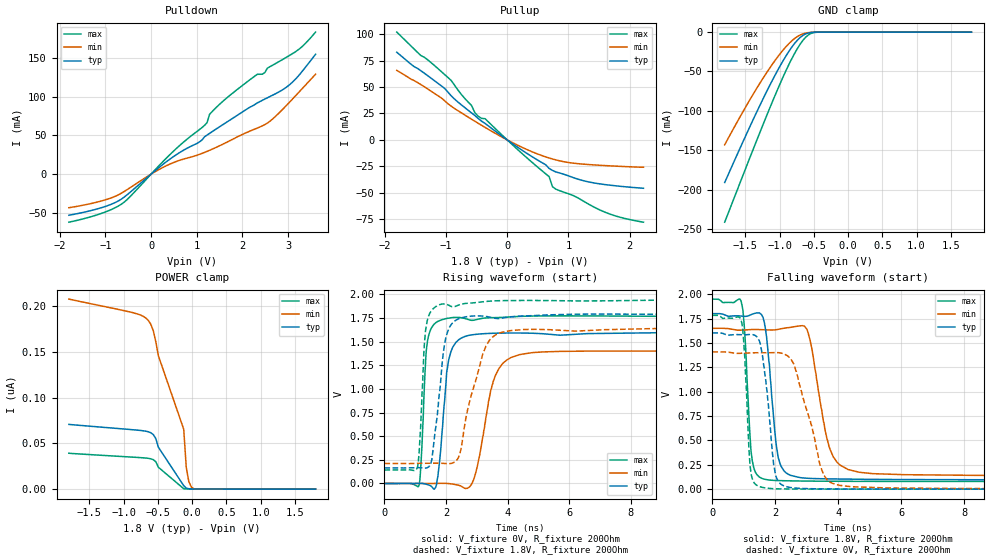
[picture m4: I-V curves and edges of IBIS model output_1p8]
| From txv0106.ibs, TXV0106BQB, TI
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|   io_1p8 Model
[Model]   output_1p8
Model_type   I/O
Polarity   Non-Inverting
Enable   Active-High
Vinl = 0.54
Vinh = 1.26
Vmeas = 0.9
Vref = 0
Cref = 2pF
Rref = 100000
|   typ   min   max
C_comp   1.540pF   1.379pF   1.785pF
| Where Nom  PVT is Nominal Process, 1.8V,  27C
|   Fast PVT is Strong Process,  1.95V, -40C
|   Slow PVT is Weak Process,   1.65V, 125C
[Voltage Range]   1.8   1.65   1.95
|Junction Temperature
[Temperature Range]   27   125   -40
[Pullup Reference]   1.8   1.65   1.95
[Pulldown Reference]   0   0   0
[Power Clamp Reference]   1.8   1.65   1.95
[GND Clamp Reference]   0   0   0
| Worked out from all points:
|   slope of the pulldown table from 0 to 0.27 V, typ, clamps not added: 20.6 ohm
|   slope of the pullup table from 0 to 0.27 V, typ, clamps not added: 24.9 ohm
|   GND clamp passes 1 mA (typ) near -0.57 V on its own axis
|   falling waveform, V_fixture 1.8V, R_fixture 200Ohm: 20-80 % time 283ps typ, 502ps min, 181ps max; typ from 1.8 V to 0.095 V
|   rising waveform, V_fixture 0V, R_fixture 200Ohm: 20-80 % time 257ps typ, 502ps min, 155ps max; typ from 0 V to 1.6 V
|   rising waveform, V_fixture 1.8V, R_fixture 200Ohm: 20-80 % time 329ps typ, 637ps min, 169ps max; typ from 0.165 V to 1.8 V
|   falling waveform, V_fixture 0V, R_fixture 200Ohm: 20-80 % time 301ps typ, 667ps min, 160ps max; typ from 1.6 V to 0 V
[Pulldown]
|Voltage   I(typ)   I(min)   I(max)
-1.8V     -53.1mA    -43.34mA   -62.05mA
-1.03V    -42.27mA   -33.68mA   -49.51mA
-590mV    -29.71mA   -22.47mA   -36.17mA
345mV     16.5mA     11.18mA    21.32mA
1.17V     48.16mA    28.03mA    62.98mA
1.225V    50.41mA    29.37mA    66.56mA
1.28V     52.62mA    30.75mA    77.23mA
1.5V      61.19mA    36.66mA    90.28mA
2.325V    91.98mA    59.5mA     128.9mA
2.49V     96.93mA    63.94mA    131.2mA
3.04V     115.9mA    93.53mA    153.6mA
3.6V      154.8mA    129mA      183.4mA
[GND Clamp]
|Voltage   I(typ)   I(min)   I(max)
-1.8V     -191mA     -143.1mA   -241.4mA
-1.578V   -147.8mA   -107.9mA   -191.8mA
-1.356V   -105.8mA   -74.75mA   -142.6mA
-1.171V   -72.59mA   -49.3mA    -102.6mA
-986mV    -42.13mA   -26.9mA    -64.4mA
-875mV    -26.05mA   -15.67mA   -43.28mA
-764mV    -12.71mA   -7.063mA   -24.62mA
-653mV    -3.853mA   -2.076mA   -9.887mA
-579mV    -1.121mA   -675.7uA   -3.576mA
-505mV    -223.2uA   -170.7uA   -768.7uA
-394mV    -11.53uA   -14.74uA   -30.66uA
1.8V      0A         0A         0A
[Pullup]
|Voltage   I(typ)   I(min)   I(max)
-1.8V     83.07mA    65.91mA    102.2mA
-1.405V   65.45mA    52.34mA    79.85mA
-1.02V    48.82mA    37.12mA    61.96mA
-910mV    41.62mA    31.84mA    56.13mA
-580mV    25.53mA    19.56mA    32.63mA
-525mV    23.02mA    17.6mA     25.57mA
-195mV    8.317mA    6.238mA    10.81mA
685mV     -27.1mA    -17.21mA   -34.82mA
740mV     -29mA      -18.16mA   -44.48mA
1.235V    -38.6mA    -23.01mA   -57.78mA
1.62V     -42.6mA    -24.48mA   -69.16mA
2.225V    -45.93mA   -25.97mA   -78.1mA
[POWER Clamp]
|Voltage   I(typ)   I(min)   I(max)
-1.8V     70.75nA    207.7nA    39.26nA
-790mV    64.4nA     191.2nA    34.62nA
-679mV    63.35nA    187.1nA    34.01nA
-605mV    61.67nA    180.3nA    33.2nA
-568mV    59.62nA    173.1nA    32.21nA
-531mV    55.25nA    161nA      29.88nA
-494mV    45.84nA    145.8nA    23.95nA
-124mV    3.805nA    65.43nA    485.7pA
-87mV     1.147nA    23.84nA    235.2pA
-50mV     439pA      8.249nA    184.2pA
-13mV     246.6pA    2.405nA    165pA
1.8V      0A         0A         0A
[Ramp]
R_load = 200
|   typ   min   max
dV/dt_r   0.962/0.256n   0.845/0.506n   1.070/0.155n
dV/dt_f   1.023/0.282n   0.912/0.507n   1.123/0.180n
[Falling Waveform]
V_fixture = 1.8V
V_fixture_min = 1.65V
V_fixture_max = 1.95V
R_fixture = 200Ohm
C_fixture = 0F
|Time   V(typ)   V(min)   V(max)
0s        1.8V       1.65V      1.95V
910ps     1.776V     1.632V     1.931V
1.02ns    1.773V     1.633V     1.646V
1.23ns    1.79V      1.637V     385mV
1.61ns    1.762V     1.635V     106.3mV
2.12ns    297.4mV    1.642V     87.89mV
3ns       112.4mV    1.642V     83mV
3.96ns    104.4mV    276.9mV    80.94mV
6.12ns    98.55mV    148.5mV    79.3mV
200ns     94.71mV    129.3mV    78.59mV
[Rising Waveform]
V_fixture = 0V
V_fixture_min = 0V
V_fixture_max = 0V
R_fixture = 200Ohm
C_fixture = 0F
|Time   V(typ)   V(min)   V(max)
0s        8.016uV    8.514uV    7.961uV
1.13ns    1.528mV    56.81uV    -13.27mV
1.37ns    -9.537mV   -93.25uV   1.435V
1.66ns    -44.15mV   521.7uV    1.697V
2.03ns    1.19V      257.3uV    1.745V
2.32ns    1.49V      -12.58mV   1.756V
2.88ns    1.573V     25.06mV    1.725V
3.85ns    1.59V      1.271V     1.756V
5.71ns    1.567V     1.396V     1.772V
200ns     1.603V     1.408V     1.784V
[Rising Waveform]
V_fixture = 1.8V
V_fixture_min = 1.65V
V_fixture_max = 1.95V
R_fixture = 200Ohm
C_fixture = 0F
|Time   V(typ)   V(min)   V(max)
0s        164.6mV    211.2mV    142.3mV
1.08ns    167.1mV    213.2mV    181.3mV
1.3ns     162.2mV    213.3mV    1.483V
1.51ns    212.3mV    213.8mV    1.819V
1.91ns    1.372V     211.9mV    1.898V
2.11ns    1.648V     209.2mV    1.881V
2.45ns    1.745V     312mV      1.891V
3.18ns    1.77V      1.352V     1.92V
3.69ns    1.743V     1.584V     1.932V
200ns     1.8V       1.65V      1.95V
[Falling Waveform]
|Gnd
V_fixture = 0V
V_fixture_min = 0V
V_fixture_max = 0V
R_fixture = 200Ohm
C_fixture = 0F
|   Time   V(typ)   V(min)   V(max)
0s        1.603V     1.408V     1.784V
920ps     1.584V     1.394V     1.723V
1.03ns    1.583V     1.396V     1.354V
1.21ns    1.587V     1.398V     208.2mV
1.49ns    1.523V     1.4V       27.9mV
2.05ns    107.6mV    1.401V     3.585mV
2.59ns    12.48mV    1.281V     1.456mV
3.64ns    2.435mV    97.98mV    552.1uV
5.54ns    850.1uV    12.54mV    220.9uV
200ns     -724.3nV   12.17uV    -6.005nV
